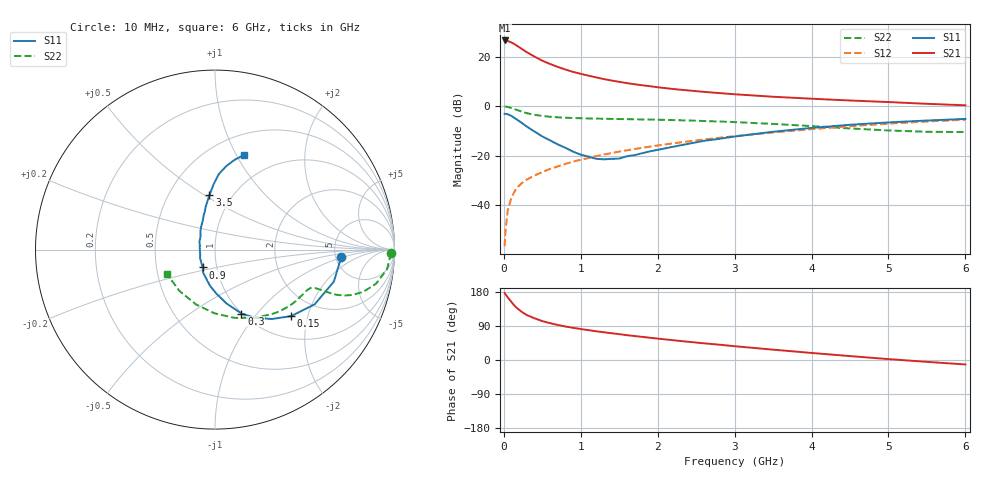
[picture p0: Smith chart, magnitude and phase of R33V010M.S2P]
! SIEMENS Small Signal Semiconductors
! BFR181
! Si NPN RF Bipolar Junction Transistor in SOT23
! VCE = 3 V  IC = 10 mA
! Common Emitter S-Parameters:  May  1996
# GHz  S  MA  R  50
!  f  S11  S21  S12  S22
! GHz  MAG  ANG  MAG  ANG  MAG  ANG  MAG  ANG
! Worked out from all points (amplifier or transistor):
!   36 points, 10 MHz to 6 GHz, reference 50 ohm
!   highest |S21| = 26.5 dB at 10 MHz (marker M1)
!   |S21| within 3 dB of that: start of sweep to 213.1 MHz
!   unconditionally stable (mu >= 1): 755.2 MHz to 2.65 GHz
!   at 250 MHz: K = 0.61, MSG = 26.7 dB, |S12| = -30.6 dB
!   at 1.4 GHz: K = 1.07, MAG = 13.1 dB, |S12| = -19.0 dB
!   at 6 GHz: K = 0.85, MSG = 2.9 dB, |S12| = -5.5 dB
!   S11 on the Smith chart (normalised r, x): 10 MHz: 5.63, -0.88; 150 MHz: 1.45, -1.58; 300 MHz: 1.00, -0.83; 900 MHz: 0.86, -0.17; 3.5 GHz: 0.79, +0.52; 6 GHz: 0.71, +1.08
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0.01  0.7045 -3.2  21.12 176.8  0.0015 91.7  0.9829 -1.2
0.02  0.6977 -6.1  20.97 173.8  0.0029 82.5  0.9756 -2.6
0.05  0.6857 -15.1  20.64 165.6  0.0078 80.5  0.9649 -6.5
0.1  0.6333 -28.8  19.19 152.7  0.0145 78.4  0.9177 -11.9
0.15  0.5629 -41.2  17.3 140.7  0.0204 72.9  0.8592 -15.9
0.2  0.4997 -50.7  15.42 132.1  0.025 70.0  0.8055 -18.3
0.25  0.4394 -59.8  13.7 124.6  0.0294 68.1  0.7591 -19.7
0.3  0.3854 -67.5  12.21 118.5  0.0331 68.3  0.721 -20.4
0.4  0.3067 -78.0  9.945 110.0  0.04 67.7  0.6675 -20.8
0.5  0.2449 -88.3  8.252 102.7  0.0468 68.6  0.6337 -20.8
0.6  0.2043 -97.6  7.085 97.2  0.0542 68.8  0.6108 -20.9
0.7  0.1695 -106.6  6.194 92.5  0.0608 69.7  0.5956 -21.0
0.9  0.1209 -124.5  4.908 84.9  0.076 69.9  0.5762 -21.7
1.1  0.0961 -150.5  4.118 78.8  0.0902 70.2  0.5646 -23.1
1.3  0.0845 -175.2  3.513 73.2  0.1058 69.7  0.5564 -24.8
1.6  0.0976 152.6  2.912 65.5  0.1287 69.0  0.5464 -28.0
2.2  0.1517 120.2  2.215 52.2  0.1775 65.9  0.5234 -35.9
2.8  0.2193 104.9  1.834 40.4  0.2297 61.5  0.4904 -45.6
3.5  0.3039 95.9  1.547 27.3  0.2947 55.2  0.4381 -60.2
4.5  0.4212 87.1  1.3 10.3  0.3942 44.2  0.3553 -90.4
5.5  0.513 77.6  1.114 -4.9  0.4905 31.1  0.3039 -130.5
6  0.5522 72.8  1.04 -11.8  0.5334 24.0  0.3002 -152.6
